//DB985.AWL
// ***************************************************************************


DATA_BLOCK "XC_JOB_SR"
TITLE = Cross Coupling jobs

AUTHOR: 	SIEMENS
FAMILY: 	SISTARS7
NAME:		XCJOBDBSR
VERSION: 	4.02

//$NOW_HOW_PROTECT

//
// Datum		Name			Aktion
// ----------------------------------------------------------------------------
// 19.05.99 	Mahler		Neu

  STRUCT

	iType			: INT		:= 1;
   	iOffset 		: INT  	:= 3604;  //Anfang von Wegest. + Anwender dh. 64*56+20
   	iLen 			: INT  	:= 56;


//#IF Default
   	iMax 			: INT  	:= 256;	//64 Wegest. + 192 Anwender
   	iAct 			: INT  	:= 256;
//#ENDIF

//#IF Special
// 	iMax 			: INT  	:= %XC_JOB_USR%;
// 	iAct 			: INT  	:= %XC_JOB_USR%;
//#ENDIF

   	iSys			: INT		:= 64;			//ASTA + System
	iOffsetSys		: INT		:= 20;

//#IF Default
	iActSum		: INT		:= 320;			//iSys + iAct max. 320 je kleiner je besser
//#ENDIF

//#IF Special
//	iActSum		: INT		:= %XC_JOB_SUM%;	//iSys + iAct
//#ENDIF

	iNumPerSrch	: INT		:= 50;			//Datensätze je Suche
	w			: WORD;

	auSys			: ARRAY [1..64] OF "XC_JOB_SR_UDT"; //ASTA + System

//#IF Default
	au			: ARRAY [1..256] OF "XC_JOB_SR_UDT"; //64 Wegest. + xx Anwender
//#ENDIF

//#IF Special
//	au			: ARRAY [1..%XC_JOB_USR%] OF "XC_JOB_SR_UDT";
//#ENDIF




END_STRUCT ;

BEGIN

END_DATA_BLOCK

